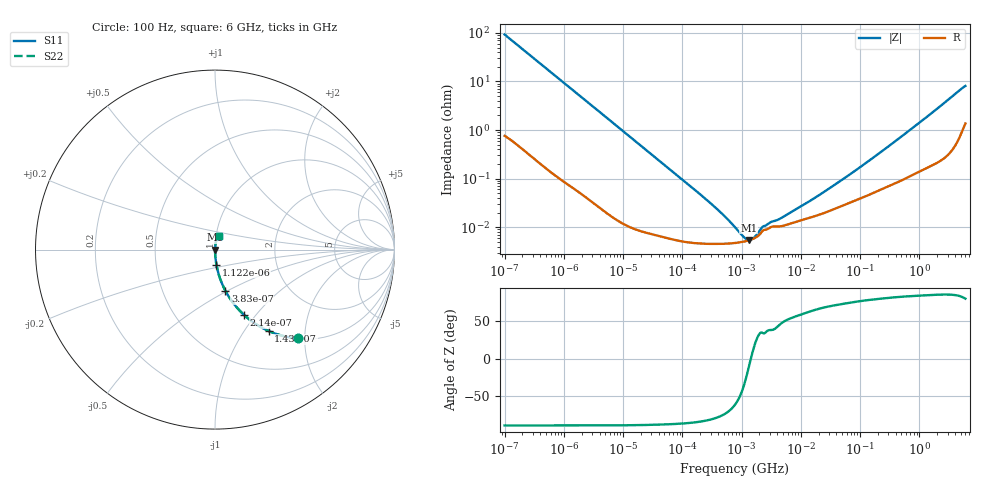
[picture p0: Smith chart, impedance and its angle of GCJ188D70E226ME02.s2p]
!Murata Part Number: GCJ188D70E226ME02
!These Parameters are Measured in Series Mode Connection
!Data Generated on Mar 13, 2026
!  o--ll--o
!Port1  Port2
!  o------o
!Operation Temp=25[degC], DC Bias Voltage=0[V]
!Freq. Start=100[Hz] Stop=6[GHz] 401[Steps]
# Hz S RI R 50
!Freq.(Hz) S11(Real) S11(Imag) S21(Real) S21(Imag) S12(Real) S12(Imag) S22(Real) S22(Imag)
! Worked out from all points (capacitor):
!   401 points, 100 Hz to 6 GHz, reference 50 ohm
!   read as one part in series: C = 17.1 uF near 109 Hz
!   lowest |Z| = 5.49 mohm at 1.326 MHz (marker M1)
!   series resonance near 1.436 MHz, so ESL is about 720 pH
!   S11 on the Smith chart (normalised r, x): 100 Hz: 1.02, -1.85; 143 Hz: 1.01, -1.30; 214 Hz: 1.01, -0.87; 383 Hz: 1.00, -0.49; 1.122 kHz: 1.00, -0.17; 6 GHz: 1.03, +0.16
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100  0.4625 -0.4945  0.5375 0.4945  0.5375 0.4945  0.4625 -0.4945
143  0.2983 -0.4532  0.7017 0.4532  0.7017 0.4532  0.2983 -0.4532
214  0.1614 -0.3636  0.8386 0.3636  0.8386 0.3636  0.1614 -0.3636
383  0.0579 -0.2293  0.9421 0.2293  0.9421 0.2293  0.0579 -0.2293
627  0.0231 -0.1458  0.9769 0.1458  0.9769 0.1458  0.0231 -0.1458
1122  0.00773 -0.083  0.9923 0.083  0.9923 0.083  0.00773 -0.083
2008  0.00267 -0.0468  0.9973 0.0468  0.9973 0.0468  0.00267 -0.0468
6433  0.000383 -0.0148  0.9996 0.0148  0.9996 0.0148  0.000383 -0.0148
40335  7.16e-05 -0.00237  0.9999 0.00237  0.9999 0.00237  7.16e-05 -0.00237
276587  4.57e-05 -0.000337  1 0.000337  1 0.000337  4.57e-05 -0.000337
774597  4.75e-05 -8.84e-05  1 8.84e-05  1 8.84e-05  4.75e-05 -8.84e-05
1325623  5.38e-05 -1.07e-05  0.9999 1.07e-05  0.9999 1.07e-05  5.38e-05 -1.07e-05
1983483  6.95e-05 4.46e-05  0.9999 -4.46e-05  0.9999 -4.46e-05  6.95e-05 4.46e-05
2372521  8.79e-05 5.85e-05  0.9999 -5.85e-05  0.9999 -5.85e-05  8.79e-05 5.85e-05
3103719  0.0001 7.91e-05  0.9999 -7.91e-05  0.9999 -7.91e-05  0.0001 7.91e-05
4643984  0.000105 0.000113  0.9999 -0.000113  0.9999 -0.000113  0.000105 0.000113
1.555665e7  0.000163 0.000334  0.9998 -0.000334  0.9998 -0.000334  0.000163 0.000334
6.817316e7  0.000322 0.00119  0.9997 -0.00119  0.9997 -0.00119  0.000322 0.00119
3.124326e8  0.00073 0.00471  0.9993 -0.00471  0.9993 -0.00471  0.00073 0.00471
1.791126e9  0.00257 0.0245  0.9974 -0.0245  0.9974 -0.0245  0.00257 0.0245
4.796499e9  0.0113 0.0646  0.9887 -0.0646  0.9887 -0.0646  0.0113 0.0646
6e9  0.0195 0.0771  0.9805 -0.0771  0.9805 -0.0771  0.0195 0.0771
